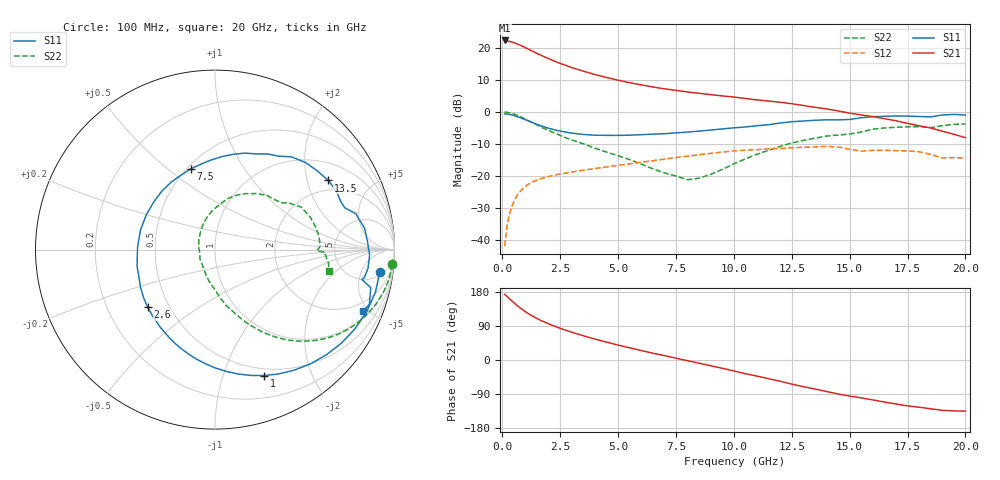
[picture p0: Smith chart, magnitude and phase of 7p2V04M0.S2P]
! Infineon Technologies  Discrete & RF Semiconductors
! bfp620
! VCE =  2.0 V,  IC =  4.0 mA
! Common Emitter S-Parameters:  Sep 2002
# GHz  S  MA  R  50
!  f  S11  S21  S12  S22
! GHz  MAG  ANG  MAG  ANG  MAG  ANG  MAG  ANG
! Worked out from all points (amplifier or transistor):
!   59 points, 100 MHz to 20 GHz, reference 50 ohm
!   highest |S21| = 22.3 dB at 100 MHz (marker M1)
!   |S21| within 3 dB of that: start of sweep to 1.206 GHz
!   unconditionally stable (mu >= 1): 5.048 GHz to 11.93 GHz; 14.55 GHz to 15.45 GHz; 17.24 GHz to end of sweep
!   at 1 GHz: K = 0.27, MSG = 21.6 dB, |S12| = -23.3 dB
!   at 5.5 GHz: K = 1.04, MAG = 11.5 dB, |S12| = -16.2 dB
!   at 20 GHz: K = 1.34, MAG = -0.3 dB, |S12| = -14.4 dB
!   S11 on the Smith chart (normalised r, x): 100 MHz: 6, -11; 1 GHz: 0.42, -1.38; 2.6 GHz: 0.38, -0.32; 7.5 GHz: 0.52, +0.60; 13.5 GHz: 1.59, +2.71; 20 GHz: 1.35, -4.60
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0.1  0.9266 -7.7  13.02 173.5  0.008 80.6  0.9912 -4.8
0.2  0.9249 -14.9  12.86 167.9  0.0163 80.7  0.9838 -9.4
0.4  0.8962 -29.5  12.32 156.5  0.0324 73.8  0.9481 -18.5
0.6  0.8533 -43.5  11.64 145.8  0.0467 66.5  0.8956 -26.9
0.8  0.8046 -56.5  10.87 136.1  0.0588 59.9  0.8345 -34.3
1  0.7537 -68.6  10.04 127.5  0.0687 54.0  0.7703 -40.7
1.3  0.6808 -84.9  8.864 116.1  0.0803 46.8  0.678 -48.6
1.7  0.6013 -104.0  7.559 103.5  0.0914 39.8  0.5745 -56.6
2.2  0.5307 -124.6  6.308 90.6  0.1017 33.7  0.4758 -64.1
2.6  0.4935 -139.5  5.531 81.5  0.1086 30.0  0.4132 -69.1
3  0.4651 -153.1  4.916 73.3  0.115 26.8  0.3638 -73.4
3.5  0.4438 -168.1  4.316 63.9  0.1229 23.4  0.3175 -78.6
5  0.429 153.3  3.12 39.4  0.1462 14.7  0.2067 -93.4
6  0.4403 132.3  2.638 25.0  0.1635 8.9  0.1529 -108.6
7  0.4561 114.3  2.289 11.6  0.1826 2.8  0.1114 -128.5
7.5  0.4701 106.6  2.167 4.8  0.1938 -1.0  0.0994 -147.2
8.5  0.5006 92.2  1.95 -8.4  0.2141 -8.6  0.0922 170.5
10.5  0.5807 66.6  1.617 -36.2  0.2519 -28.0  0.1844 104.3
12  0.6698 50.5  1.41 -56.1  0.2675 -41.7  0.2901 76.7
13.5  0.7393 31.4  1.179 -76.5  0.2835 -57.2  0.3882 53.5
17  0.8619 -2.1  0.726 -116.2  0.2481 -88.0  0.5744 12.8
20  0.893 -22.7  0.396 -134.9  0.1904 -103.5  0.6453 -10.8
